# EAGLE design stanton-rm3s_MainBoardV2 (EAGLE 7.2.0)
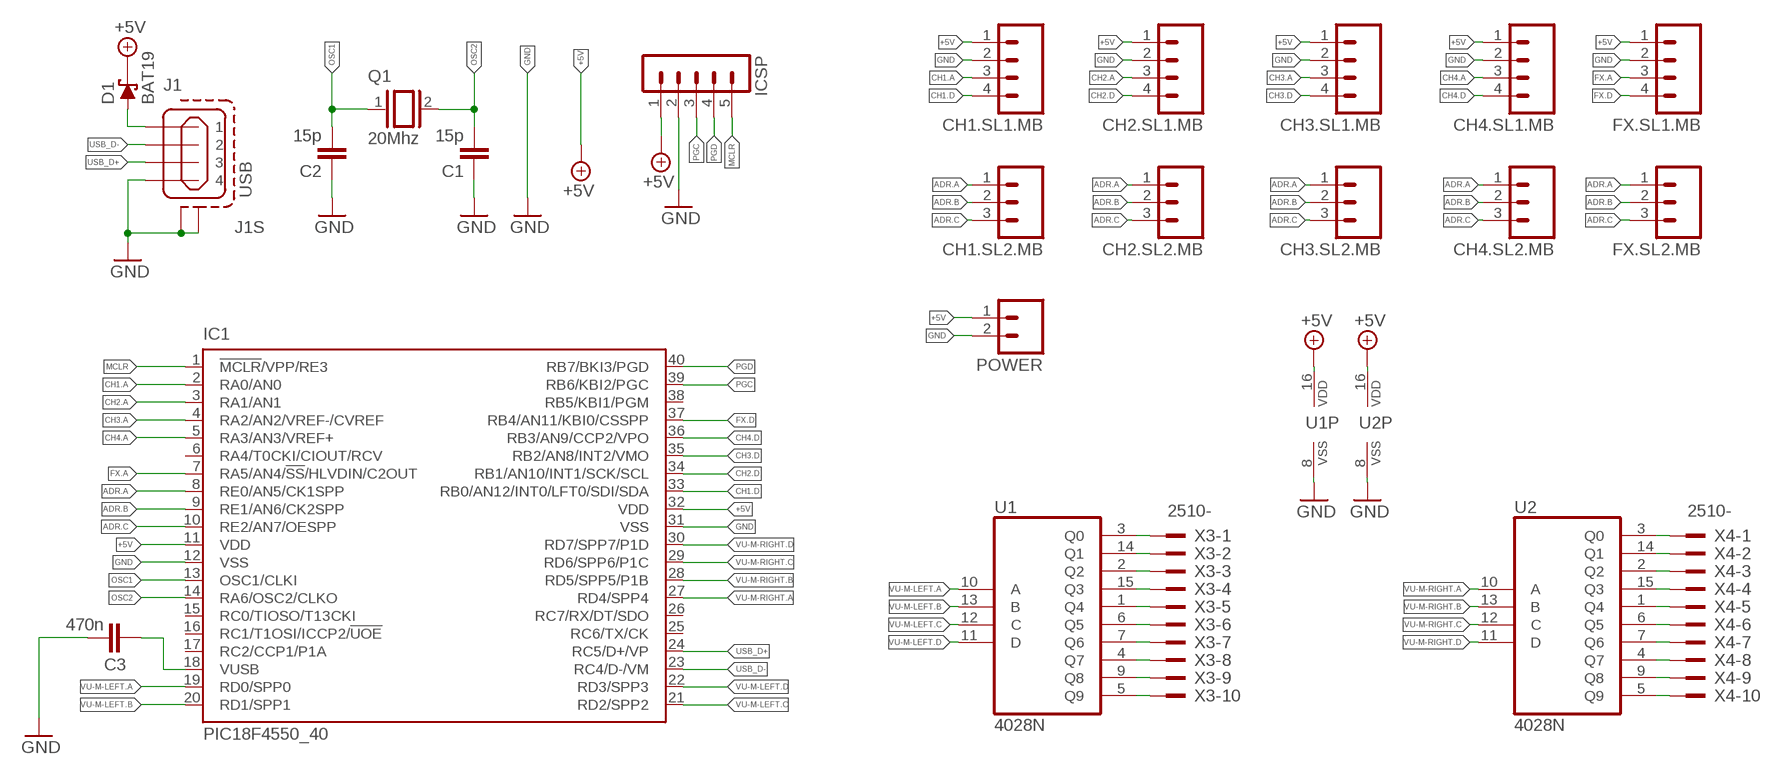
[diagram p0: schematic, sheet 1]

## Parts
C1  15p  C-EU050-024X044  [C050-024X044]
C2  15p  C-EU050-024X044  [C050-024X044]
C3  470n  C-EU050-024X044  [C050-024X044]
CH1.SL1.MB  M04  [04P]
CH1.SL2.MB  M03  [03P]
CH2.SL1.MB  M04  [04P]
CH2.SL2.MB  M03  [03P]
CH3.SL1.MB  M04  [04P]
CH3.SL2.MB  M03  [03P]
CH4.SL1.MB  M04  [04P]
CH4.SL2.MB  M03  [03P]
D1  BAT19  [DO35-10]
FX.SL1.MB  M04  [04P]
FX.SL2.MB  M03  [03P]
IC1  PIC18F4550_40  [DIL40]
ICSP  MA05-1  [MA05-1]
J1  USB  MINI-USB_SHIELD4P-85-32004-00X  [85-32004-00X]
POWER  M02  [02P]
Q1  20Mhz  XTAL/S  [QS]
U1  4028N  [DIL16]
U2  4028N  [DIL16]
X3  2510-  [PAK100/2500-10]
X4  2510-  [PAK100/2500-10]

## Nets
+5V: CH1.SL1.MB.1 CH2.SL1.MB.1 CH3.SL1.MB.1 CH4.SL1.MB.1 D1.C FX.SL1.MB.1 IC1.11(VDD) IC1.32(VDD) ICSP.1 POWER.1 U1.16(VDD) U2.16(VDD)
ADR.A: CH1.SL2.MB.1 CH2.SL2.MB.1 CH3.SL2.MB.1 CH4.SL2.MB.1 FX.SL2.MB.1 IC1.8(RE0/AN5/CK1SPP)
ADR.B: CH1.SL2.MB.2 CH2.SL2.MB.2 CH3.SL2.MB.2 CH4.SL2.MB.2 FX.SL2.MB.2 IC1.9(RE1/AN6/CK2SPP)
ADR.C: CH1.SL2.MB.3 CH2.SL2.MB.3 CH3.SL2.MB.3 CH4.SL2.MB.3 FX.SL2.MB.3 IC1.10(RE2/AN7/OESPP)
CH1.A: CH1.SL1.MB.3 IC1.2(RA0/AN0)
CH1.D: CH1.SL1.MB.4 IC1.33(RB0/AN12/INT0/LFT0/SDI/SDA)
CH2.A: CH2.SL1.MB.3 IC1.3(RA1/AN1)
CH2.D: CH2.SL1.MB.4 IC1.34(RB1/AN10/INT1/SCK/SCL)
CH3.A: CH3.SL1.MB.3 IC1.4(RA2/AN2/VREF-/CVREF)
CH3.D: CH3.SL1.MB.4 IC1.35(RB2/AN8/INT2/VMO)
CH4.A: CH4.SL1.MB.3 IC1.5(RA3/AN3/VREF+)
CH4.D: CH4.SL1.MB.4 IC1.36(RB3/AN9/CCP2/VPO)
FX.A: FX.SL1.MB.3 IC1.7(RA5/AN4/!SS!/HLVDIN/C2OUT)
FX.D: FX.SL1.MB.4 IC1.37(RB4/AN11/KBI0/CSSPP)
GND: C1.1 C2.1 C3.1 CH1.SL1.MB.2 CH2.SL1.MB.2 CH3.SL1.MB.2 CH4.SL1.MB.2 FX.SL1.MB.2 IC1.12(VSS) IC1.31(VSS) ICSP.2 J1.4 J1.M1(S1) J1.M2(S2) POWER.2 U1.8(VSS) U2.8(VSS)
MCLR: IC1.1(!MCLR!/VPP/RE3) ICSP.5
N$5: C3.2 IC1.18(VUSB)
N$29: D1.A J1.1
N$57: U1.3(Q0) X3.1
N$58: U1.14(Q1) X3.2
N$59: U1.2(Q2) X3.3
N$60: U1.15(Q3) X3.4
N$61: U1.1(Q4) X3.5
N$62: U1.6(Q5) X3.6
N$63: U1.7(Q6) X3.7
N$64: U1.4(Q7) X3.8
N$65: U1.9(Q8) X3.9
N$66: U1.5(Q9) X3.10
N$67: U2.3(Q0) X4.1
N$68: U2.14(Q1) X4.2
N$69: U2.2(Q2) X4.3
N$70: U2.15(Q3) X4.4
N$71: U2.1(Q4) X4.5
N$72: U2.6(Q5) X4.6
N$73: U2.7(Q6) X4.7
N$74: U2.4(Q7) X4.8
N$75: U2.9(Q8) X4.9
N$76: U2.5(Q9) X4.10
OSC1: C2.2 IC1.13(OSC1/CLKI) Q1.1
OSC2: C1.2 IC1.14(RA6/OSC2/CLKO) Q1.2
PGC: IC1.39(RB6/KBI2/PGC) ICSP.3
PGD: IC1.40(RB7/BKI3/PGD) ICSP.4
USB_D+: IC1.24(RC5/D+/VP) J1.3
USB_D-: IC1.23(RC4/D-/VM) J1.2
VU-M-LEFT.A: IC1.19(RD0/SPP0) U1.10(A)
VU-M-LEFT.B: IC1.20(RD1/SPP1) U1.13(B)
VU-M-LEFT.C: IC1.21(RD2/SPP2) U1.12(C)
VU-M-LEFT.D: IC1.22(RD3/SPP3) U1.11(D)
VU-M-RIGHT.A: IC1.27(RD4/SPP4) U2.10(A)
VU-M-RIGHT.B: IC1.28(RD5/SPP5/P1B) U2.13(B)
VU-M-RIGHT.C: IC1.29(RD6/SPP6/P1C) U2.12(C)
VU-M-RIGHT.D: IC1.30(RD7/SPP7/P1D) U2.11(D)
Unconnected: IC1.6(RA4/T0CKI/CIOUT/RCV) IC1.15(RC0/TIOSO/T13CKI) IC1.16(RC1/T1OSI/ICCP2/!UOE) IC1.17(RC2/CCP1/P1A) IC1.25(RC6/TX/CK) IC1.26(RC7/RX/DT/SDO) IC1.38(RB5/KBI1/PGM)

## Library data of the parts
C1-C3 = resistor:C-EU: CAPACITOR, European symbol
CH1.SL1.MB CH2.SL1.MB CH3.SL1.MB CH4.SL1.MB FX.SL1.MB = con-amp-quick:M04: AMP QUICK CONNECTOR
CH1.SL2.MB CH2.SL2.MB CH3.SL2.MB CH4.SL2.MB FX.SL2.MB = con-amp-quick:M03: AMP QUICK CONNECTOR
D1 = diode:BAT19: DIODE
IC1 = microchip:PIC18F4*_40: USB Microcontrollers with nanoWatt Technology High-Performance, Enhanced Flash, 28/40/44-Pin, Source: http://ww1.microchip.com/downloads/en/devicedoc/39632c.pdf; MF: MICROCHIP; MPN: PIC18F4550-I/P; OC_FARNELL: 9321357; OC_NEWARK: 74K8623
ICSP = con-lstb:MA05-1: PIN HEADER; OC_FARNELL: unknown; OC_NEWARK: unknown
J1 = con-cypressindustries:MINI-USB_SHIELD4P-: MINI USB 4 Pol. Source: www.cypressindustries.com
POWER = con-amp-quick:M02: AMP QUICK CONNECTOR
Q1 = special:XTAL/S: CRYSTAL
U1 U2 = 40xx:4028: BCD to decimal DECODER
X3 X4 = con-3m:2510-: 3M (TM) Pak 100 4-Wall Header Source: 3M

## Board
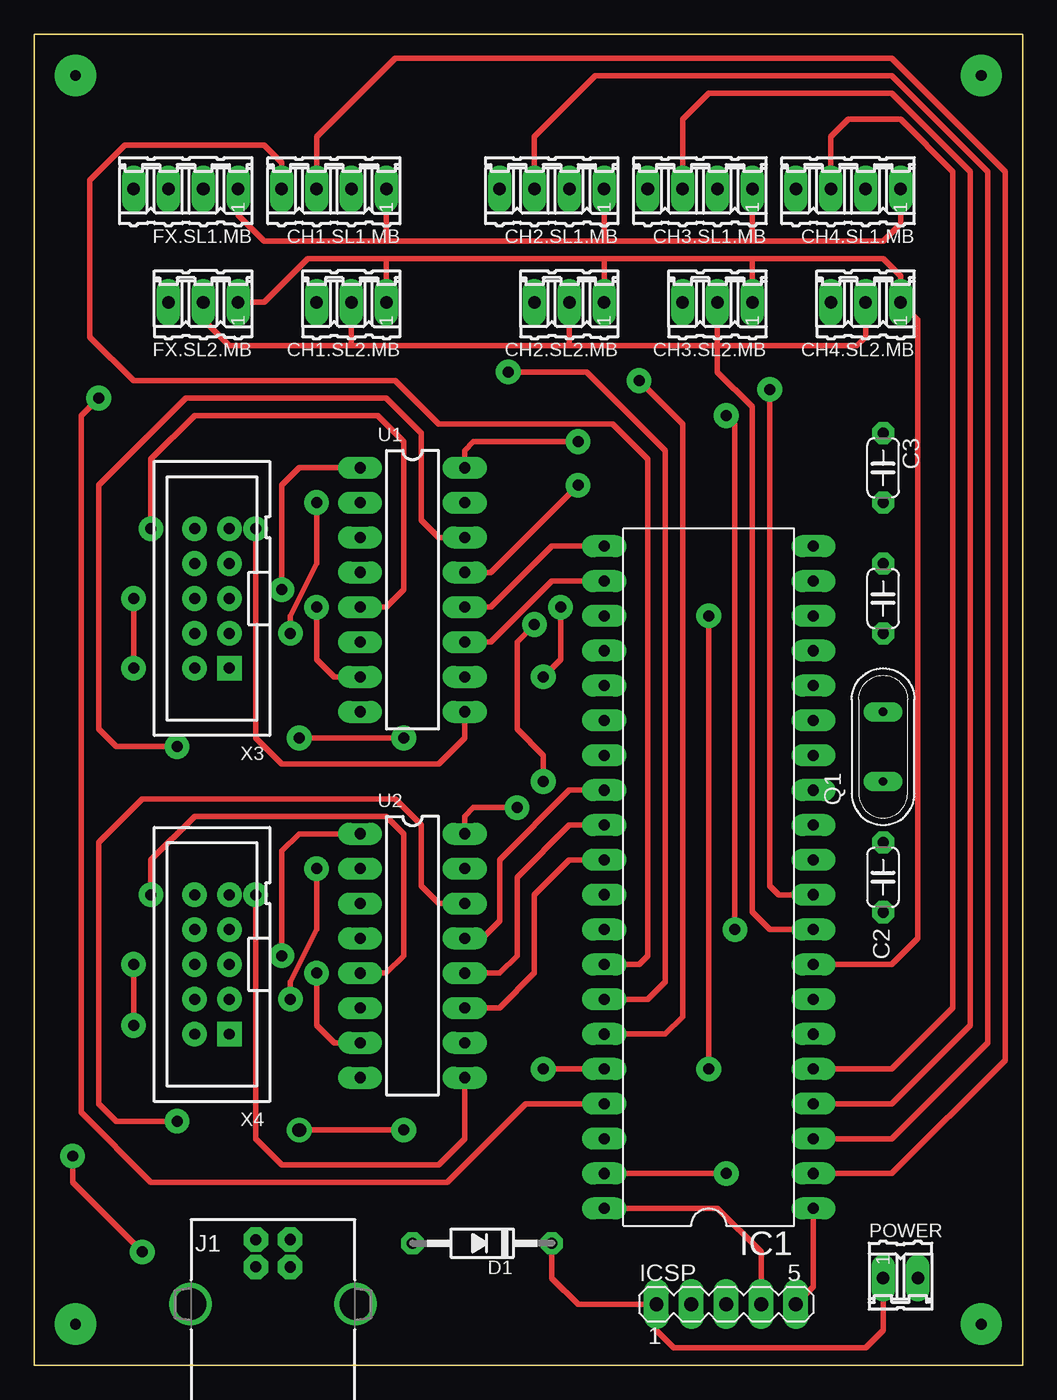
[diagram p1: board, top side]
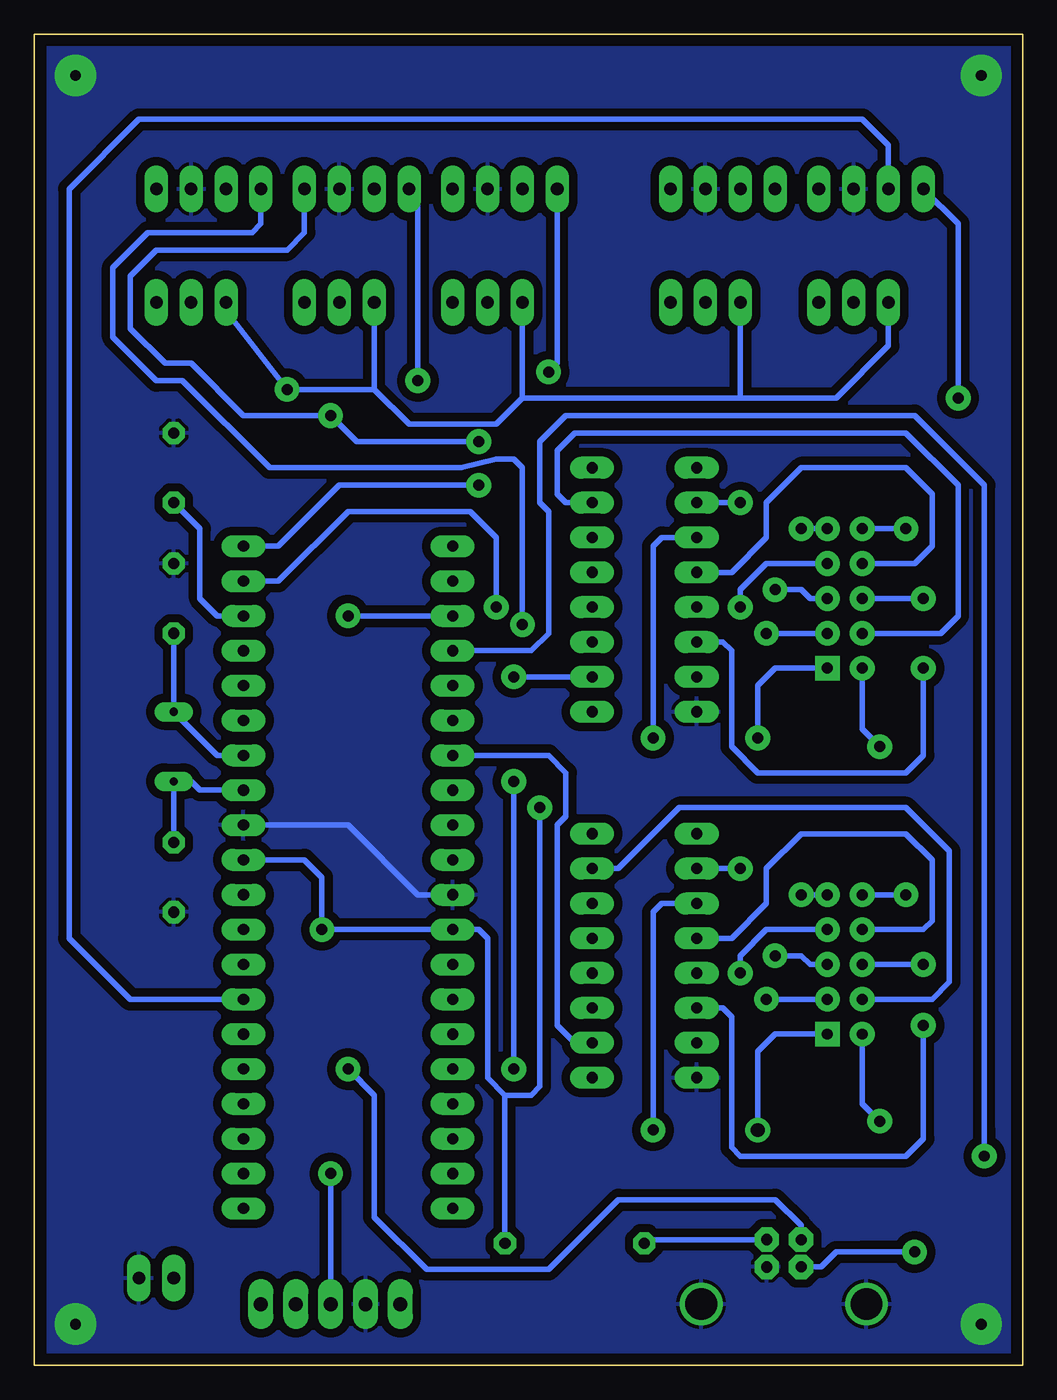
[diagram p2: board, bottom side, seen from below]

Size 72 x 97 mm. Coordinates in mm from the lower left corner, seen from the top.
Outline: 0,0 0,97 72,97 72,0 0,0
Copper layers (1*16): Top 0.035mm / dielectric 1.5mm / Bottom 0.035mm
Design rules "default *": minimum track width 0.3mm, minimum drill 0.8mm, track to track 0.4mm, track to pad 0.3mm, pad to pad 0.4mm, via to via 0.4mm, smd to smd 0.4mm, copper to edge 0.8mm, drill to drill 0.8mm, minimum pad ring 0.4mm, minimum via ring 0.2mm, stop-mask expansion 4mil, vias tented up to drill 0mil, thermal gap 10mil

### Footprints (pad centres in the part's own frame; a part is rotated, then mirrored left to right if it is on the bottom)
C050-024X044 = drill 0.813 octagon: 1 -2.54,0; 2 2.54,0
04P = drill 0.914 long: 1 -3.81,0; 2 -1.27,0; 3 1.27,0; 4 3.81,0
03P = drill 0.914 long: 1 -2.54,0; 2 0,0; 3 2.54,0
DO35-10 = drill 0.813 pad 1.524 octagon: A 5.08,0; C -5.08,0
DIL40 = drill 0.813 long: 1 -24.13,-7.62; 2 -21.59,-7.62; 3 -19.05,-7.62; 4 -16.51,-7.62; 5 -13.97,-7.62; 6 -11.43,-7.62; 7 -8.89,-7.62; 8 -6.35,-7.62; 9 -3.81,-7.62; 10 -1.27,-7.62; 11 1.27,-7.62; 12 3.81,-7.62; 13 6.35,-7.62; 14 8.89,-7.62; 15 11.43,-7.62; 16 13.97,-7.62; 17 16.51,-7.62; 18 19.05,-7.62; 19 21.59,-7.62; 20 24.13,-7.62; 21 24.13,7.62; 22 21.59,7.62; 23 19.05,7.62; 24 16.51,7.62; 25 13.97,7.62; 26 11.43,7.62; 27 8.89,7.62; 28 6.35,7.62; 29 3.81,7.62; 30 1.27,7.62; 31 -1.27,7.62; 32 -3.81,7.62; 33 -6.35,7.62; 34 -8.89,7.62; 35 -11.43,7.62; 36 -13.97,7.62; 37 -16.51,7.62; 38 -19.05,7.62; 39 -21.59,7.62; 40 -24.13,7.62
MA05-1 = drill 1.016 long: 1 -5.08,0; 2 -2.54,0; 3 0,0; 4 2.54,0; 5 5.08,0
85-32004-00X = drill 0.813 pad 1.778 octagon: 1 4.71,-1.25; 4 2.71,-1.25 | drill 0.8 pad 1.778 octagon: 2 4.71,1.25; 3 2.71,1.25 | drill 2.3 pad 3: M1 0,6.02; M2 0,-6.02
02P = drill 0.914 long: 1 -1.27,0; 2 1.27,0
QS = drill 0.61 long: 1 -2.54,0; 2 2.54,0
DIL16 = drill 0.813 long: 1 -8.89,-3.81; 2 -6.35,-3.81; 3 -3.81,-3.81; 4 -1.27,-3.81; 5 1.27,-3.81; 6 3.81,-3.81; 7 6.35,-3.81; 8 8.89,-3.81; 9 8.89,3.81; 10 6.35,3.81; 11 3.81,3.81; 12 1.27,3.81; 13 -1.27,3.81; 14 -3.81,3.81; 15 -6.35,3.81; 16 -8.89,3.81
PAK100/2500-10 = drill 0.8 pad 1.8 square: 1 -5.08,-1.27 | drill 0.8 pad 1.8: 2 -5.08,1.27; 3 -2.54,-1.27; 4 -2.54,1.27; 5 0,-1.27; 6 0,1.27; 7 2.54,-1.27; 8 2.54,1.27; 9 5.08,-1.27; 10 5.08,1.27

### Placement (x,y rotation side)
C1  61.84,55.88 270 top
C2  61.84,35.56 90 top
C3  61.84,65.41 270 top
CH1.SL1.MB  21.84,85.73 180 top
CH1.SL2.MB  23.11,77.47 180 top
CH2.SL1.MB  37.71,85.73 180 top
CH2.SL2.MB  38.98,77.47 180 top
CH3.SL1.MB  48.5,85.73 180 top
CH3.SL2.MB  49.77,77.47 180 top
CH4.SL1.MB  59.3,85.73 180 top
CH4.SL2.MB  60.57,77.47 180 top
D1  32.63,8.89 180 top
FX.SL1.MB  11.04,85.73 180 top
FX.SL2.MB  12.31,77.47 180 top
IC1  49.14,35.56 90 top
ICSP  50.41,4.45 0 top
J1  17.39,4.45 90 top
POWER  63.11,6.35 0 top
Q1  61.84,45.09 90 top
U1  27.55,56.52 270 top
U2  27.55,29.85 270 top
X3  12.94,55.88 90 top
X4  12.94,29.21 90 top

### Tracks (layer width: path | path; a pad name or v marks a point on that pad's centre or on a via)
+5V  (via drill 0.8 pad 1.8)
  Top 0.4: FX.SL1.MB.1 14.85,83.82 16.76,81.92 25.64,81.92 | 25.64,81.92 41.52,81.92 | 41.52,81.92 52.31,81.92 | 52.31,81.92 61.84,81.92 63.11,83.19 CH4.SL1.MB.1 | CH3.SL1.MB.1 52.31,81.92 | CH2.SL1.MB.1 41.52,81.92 | CH1.SL1.MB.1 25.64,81.92 | v51.04,31.75 51.04,68.58 v50.41,69.22 | D1.C 37.71,6.35 39.61,4.45 ICSP.1 45.33,2.54 46.6,1.27 | POWER.1 61.84,2.54 60.57,1.27
  Top 0.406: 60.57,1.27 46.6,1.27 | U2.16 31.36,40 32,40.64 v35.17,40.64 | U1.16 31.36,66.68 32,67.31 v39.61,67.31
  Bottom 0.4: D1.C 37.71,19.69 38.98,20.96 38.98,31.12 39.61,31.75 IC1.32 v51.04,31.75 51.04,35.56 52.31,36.83 IC1.11 | v50.41,69.22 56.76,69.22 60.57,73.03 62.47,73.03 65.02,75.57 65.02,79.38 63.11,81.28 53.59,81.28 52.31,82.55 CH3.SL1.MB.1
  Bottom 0.406: v35.17,40.64 35.17,20.32 35.8,19.69 37.71,19.69 | v39.61,67.31 48.5,67.31 v50.41,69.22
ADR.A
  Top 0.4: 41.52,80.65 52.31,80.65 | CH2.SL2.MB.1 41.52,80.65 | 25.64,80.65 CH1.SL2.MB.1 | 41.52,80.65 25.64,80.65 | FX.SL2.MB.1 16.76,77.47 19.93,80.65 25.64,80.65 | 52.31,80.65 61.84,80.65 63.11,79.38 CH4.SL2.MB.1 64.38,76.2 64.38,31.12 62.47,29.21 IC1.8 | 52.31,80.65 CH3.SL2.MB.1
ADR.B
  Top 0.4: CH3.SL2.MB.2 49.77,74.3 | 38.98,74.3 CH2.SL2.MB.2 | 49.77,74.3 38.98,74.3 | 23.11,74.3 CH1.SL2.MB.2 | 38.98,74.3 23.11,74.3 | FX.SL2.MB.2 12.31,76.2 14.21,74.3 23.11,74.3 | 49.77,74.3 59.93,74.3 60.57,74.93 CH4.SL2.MB.2 | IC1.9 53.59,31.75 52.31,33.02 52.31,69.85 49.77,72.39 49.77,74.3
ADR.C  (via drill 0.8 pad 1.8)
  Top 0.4: IC1.10 54.22,34.29 53.59,34.92 v53.59,71.12
  Bottom 0.4: 20.57,70.48 36.44,70.48 | CH1.SL2.MB.3 20.57,70.48 | FX.SL2.MB.3 9.77,74.3 13.58,70.48 20.57,70.48 | CH4.SL2.MB.3 58.03,76.84 v53.59,71.12 47.23,71.12 | 47.23,71.12 CH3.SL2.MB.3 | CH2.SL2.MB.3 36.44,70.48 | 36.44,70.48 38.34,68.58 44.7,68.58 47.23,71.12
CH1.A
  Top 0.4: CH1.SL1.MB.3 20.57,89.54 26.28,95.25 62.47,95.25 70.73,87 70.73,22.23 62.47,13.97 IC1.2
CH1.D
  Top 0.4: IC1.33 44.06,29.21 44.7,29.85 44.7,66.04 42.15,68.58 29.46,68.58 26.28,71.76 7.23,71.76 4.05,74.93 4.05,86.36 6.59,88.9 16.76,88.9 18.03,87.63 CH1.SL1.MB.4
CH2.A
  Top 0.4: CH2.SL1.MB.3 36.44,89.54 40.88,93.98 62.47,93.98 69.46,87 69.46,23.5 62.47,16.51 IC1.3
CH2.D  (via drill 0.8 pad 1.8)
  Top 0.4: IC1.34 44.7,26.67 45.96,27.94 45.96,66.68 40.25,72.39 v34.53,72.39
  Bottom 0.4: v34.53,72.39 33.9,73.03 CH2.SL1.MB.4
CH3.A
  Top 0.4: CH3.SL1.MB.3 47.23,90.81 49.14,92.71 62.47,92.71 68.19,87 68.19,24.77 62.47,19.05 IC1.4
CH3.D  (via drill 0.8 pad 1.8)
  Top 0.4: IC1.35 45.96,24.13 47.23,25.4 47.23,68.58 v44.06,71.76
  Bottom 0.4: CH3.SL1.MB.4 44.06,85.09 v44.06,71.76
CH4.A
  Top 0.4: IC1.5 62.47,21.59 66.92,26.04 66.92,87 63.11,90.81 59.3,90.81 58.03,89.54 CH4.SL1.MB.3
CH4.D  (via drill 0.8 pad 1.8)
  Top 0.4: v37.07,42.54 37.07,44.45 35.17,46.35 35.17,52.7 v36.44,53.98 | v37.07,21.59 IC1.36
  Bottom 0.4: v37.07,42.54 v37.07,21.59 | v36.44,53.98 36.44,65.41 37.07,66.04 38.34,66.04 40.88,65.41 54.85,65.41 61.2,71.76 63.11,71.76 66.29,74.93 66.29,80.01 63.74,82.55 56.12,82.55 55.49,83.19 CH4.SL1.MB.4
FX.A
  Bottom 0.4: 69.46,31.12 69.46,85.73 64.38,90.81 11.67,90.81 9.77,88.9 FX.SL1.MB.3
  Bottom 0.406: 69.46,31.12 65.02,26.67 IC1.7
FX.D  (via drill 0.8 pad 1.8)
  Top 0.406: IC1.37 35.8,19.05 30.09,13.33 8.5,13.33 3.42,18.42 3.42,69.22 v4.69,70.48
  Bottom 0.406: v4.69,70.48 4.69,83.19 FX.SL1.MB.4
GND  (via drill 0.8 pad 3)
  Bottom 0.4: IC1.12 49.14,39.37 44.06,34.29 IC1.31
  other vias: 3,3 69,3 69,94 3,94
  pour Bottom (isolate 0.61): 0.24,0.64 0.24,96.52 71.37,96.52 71.37,0.64
MCLR
  Top 0.4: IC1.1 56.76,5.71 ICSP.5
N$5
  Bottom 0.4: IC1.18 58.66,54.61 59.93,55.88 59.93,60.96 C3.2
N$29
  Bottom 0.4: J1.1 27.29,9.15 D1.A
N$57  (via drill 0.8 pad 1.8)
  Top 0.4: v19.3,45.72 v26.92,45.72
  Bottom 0.4: v26.92,45.72 26.92,59.69 26.28,60.32 U1.3 | v19.3,45.72 19.3,49.53 18.03,50.8 X3.1
N$58  (via drill 0.8 pad 1.8)
  Top 0.4: U1.14 29.46,60.32 28.19,61.59 28.19,67.95 25.64,70.48 11.04,70.48 4.69,64.14 4.69,46.35 5.96,45.09 v10.4,45.09
  Bottom 0.4: v10.4,45.09 11.67,46.35 X3.2
N$59  (via drill 0.8 pad 1.8)
  Top 0.4: v18.66,53.34 18.66,54.61 20.57,58.42 v20.57,62.86
  Bottom 0.4: v20.57,62.86 U1.2 | X3.3 v18.66,53.34
N$60
  Bottom 0.4: U1.15 33.27,62.86 33.9,63.5 33.9,66.68 32.63,67.95 8.5,67.95 4.69,64.14 4.69,54.61 5.96,53.34 X3.4
N$61  (via drill 0.8 pad 1.8)
  Top 0.4: v18.03,56.52 18.03,64.14 19.3,65.41 U1.1
  Bottom 0.4: X3.5 15.48,55.88 16.12,56.52 v18.03,56.52
N$62  (via drill 0.8 pad 1.8)
  Top 0.4: v7.23,55.88 v7.23,50.8
  Bottom 0.4: X3.6 v7.23,55.88 | U1.6 21.84,52.7 21.2,52.07 21.2,45.09 19.3,43.18 8.5,43.18 7.23,44.45 v7.23,50.8
N$63  (via drill 0.8 pad 1.8)
  Top 0.4: U1.7 21.84,50.16 20.57,51.43 v20.57,55.24
  Bottom 0.4: v20.57,55.24 20.57,56.52 18.66,58.42 X3.7
N$64
  Bottom 0.4: X3.8 7.87,58.42 6.59,59.69 6.59,63.5 8.5,65.41 16.12,65.41 18.66,62.86 18.66,60.32 21.2,57.78 U1.4
N$65  (via drill 0.8 pad 1.8)
  Top 0.4: U1.9 31.36,45.72 29.46,43.81 18.03,43.81 16.12,45.72 v16.12,60.96
  Bottom 0.4: v16.12,60.96 X3.9
N$66  (via drill 0.8 pad 1.8)
  Top 0.4: v8.5,60.96 8.5,66.04 11.67,69.22 25.01,69.22 26.92,67.31 26.92,56.52 25.64,55.24 U1.5
  Bottom 0.4: X3.10 v8.5,60.96
N$67  (via drill 0.8 pad 1.8, 1 pad 1.8)
  Top 0.4: v26.92,17.15 v19.3,17.15
  Bottom 0.4: v19.3,17.15 19.3,22.86 18.03,24.13 X4.1 | v26.92,17.15 26.92,33.02 26.28,33.66 U2.3
N$68  (via drill 0.8 pad 1.8)
  Top 0.4: U2.14 29.46,33.66 28.19,34.92 28.19,39.37 26.28,41.27 7.87,41.27 4.69,38.1 4.69,19.05 5.96,17.78 v10.4,17.78
  Bottom 0.4: X4.2 11.67,19.05 v10.4,17.78
N$69  (via drill 0.8 pad 1.8)
  Top 0.4: v18.66,26.67 18.66,27.94 20.57,31.75 v20.57,36.2
  Bottom 0.4: X4.3 v18.66,26.67 | v20.57,36.2 U2.2
N$70
  Bottom 0.4: U2.15 29.46,36.2 25.01,40.64 8.5,40.64 5.33,37.46 5.33,27.94 6.59,26.67 X4.4
N$71  (via drill 0.8 pad 1.8)
  Top 0.4: v18.03,29.85 18.03,37.46 19.3,38.73 U2.1
  Bottom 0.4: X4.5 15.48,29.21 16.12,29.85 v18.03,29.85
N$72  (via drill 0.8 pad 1.8)
  Top 0.4: v7.23,29.21 v7.23,24.77
  Bottom 0.4: X4.6 v7.23,29.21 | U2.6 21.84,26.04 21.2,25.4 21.2,15.88 20.57,15.24 8.5,15.24 7.23,16.51 v7.23,24.77
N$73  (via drill 0.8 pad 1.8)
  Top 0.4: v20.57,28.58 20.57,24.77 21.84,23.5 U2.7
  Bottom 0.4: X4.7 18.66,31.75 20.57,29.85 v20.57,28.58
N$74
  Bottom 0.4: X4.8 7.23,31.75 6.59,32.38 6.59,36.83 8.5,38.73 16.12,38.73 18.66,36.2 18.66,33.66 21.2,31.12 U2.4
N$75  (via drill 0.8 pad 1.8)
  Top 0.4: U2.9 31.36,16.51 29.46,14.61 18.03,14.61 16.12,16.51 v16.12,34.29
  Bottom 0.4: v16.12,34.29 X4.9
N$76  (via drill 0.8 pad 1.8)
  Top 0.4: U2.5 25.64,28.58 26.92,29.85 26.92,38.73 25.64,40 11.67,40 8.5,36.83 v8.5,34.29
  Bottom 0.4: v8.5,34.29 X4.10
OSC1
  Bottom 0.4: IC1.13 59.93,41.91 60.57,42.54 Q1.1 C2.2
OSC2
  Bottom 0.4: C1.2 Q1.2 58.66,44.45 IC1.14
PGC  (via drill 0.8 pad 1.8)
  Top 0.4: v50.41,13.97 IC1.39
  Bottom 0.4: ICSP.3 v50.41,13.97
PGD
  Top 0.4: IC1.40 49.77,11.43 52.95,8.26 ICSP.4
USB_D+  (via drill 0.8 pad 1.8)
  Top 0.406: v2.79,15.24 2.79,13.33 v7.87,8.26
  Bottom 0.4: 2.79,17.15 2.79,64.14 7.87,69.22 33.27,69.22 35.17,67.31 35.17,62.86 34.53,62.23 34.53,53.34 35.8,52.07 IC1.24 | 11.67,8.26 13.58,8.26 14.68,7.15 J1.3
  Bottom 0.406: 2.79,17.15 v2.79,15.24 | v7.87,8.26 11.67,8.26
USB_D-  (via drill 0.8 pad 1.8)
  Top 0.4: v49.14,21.59 v49.14,54.61
  Bottom 0.4: v49.14,54.61 IC1.23 | v49.14,21.59 47.23,19.69 47.23,10.79 43.42,6.98 34.53,6.98 29.46,12.06 18.03,12.06 16.14,10.18 J1.2
VU-M-LEFT.A  (via drill 0.8 pad 1.8)
  Top 0.4: v38.34,55.24 38.34,51.43 v37.07,50.16
  Bottom 0.4: IC1.19 54.22,57.15 49.14,62.23 40.25,62.23 38.34,60.32 v38.34,55.24 | v37.07,50.16 U1.10
VU-M-LEFT.B  (via drill 0.8 pad 1.8)
  Top 0.4: U1.13 33.27,57.78 v39.61,64.14
  Bottom 0.4: v39.61,64.14 49.77,64.14 54.22,59.69 IC1.20
VU-M-LEFT.C
  Top 0.4: IC1.21 37.71,59.69 33.27,55.24 U1.12
VU-M-LEFT.D
  Top 0.4: U1.11 33.27,52.7 37.71,57.15 IC1.22
VU-M-RIGHT.A
  Bottom 0.4: U2.10 32.63,23.5 33.9,24.77 33.9,39.37 33.27,40 33.27,43.18 34.53,44.45 IC1.27
VU-M-RIGHT.B
  Top 0.4: U2.13 32.63,31.12 33.9,32.38 33.9,36.83 38.98,41.91 IC1.28
VU-M-RIGHT.C
  Top 0.4: IC1.29 38.98,39.37 35.17,35.56 35.17,29.85 33.9,28.58 U2.12
VU-M-RIGHT.D
  Top 0.4: U2.11 33.9,26.04 36.44,28.58 36.44,34.29 38.98,36.83 IC1.30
